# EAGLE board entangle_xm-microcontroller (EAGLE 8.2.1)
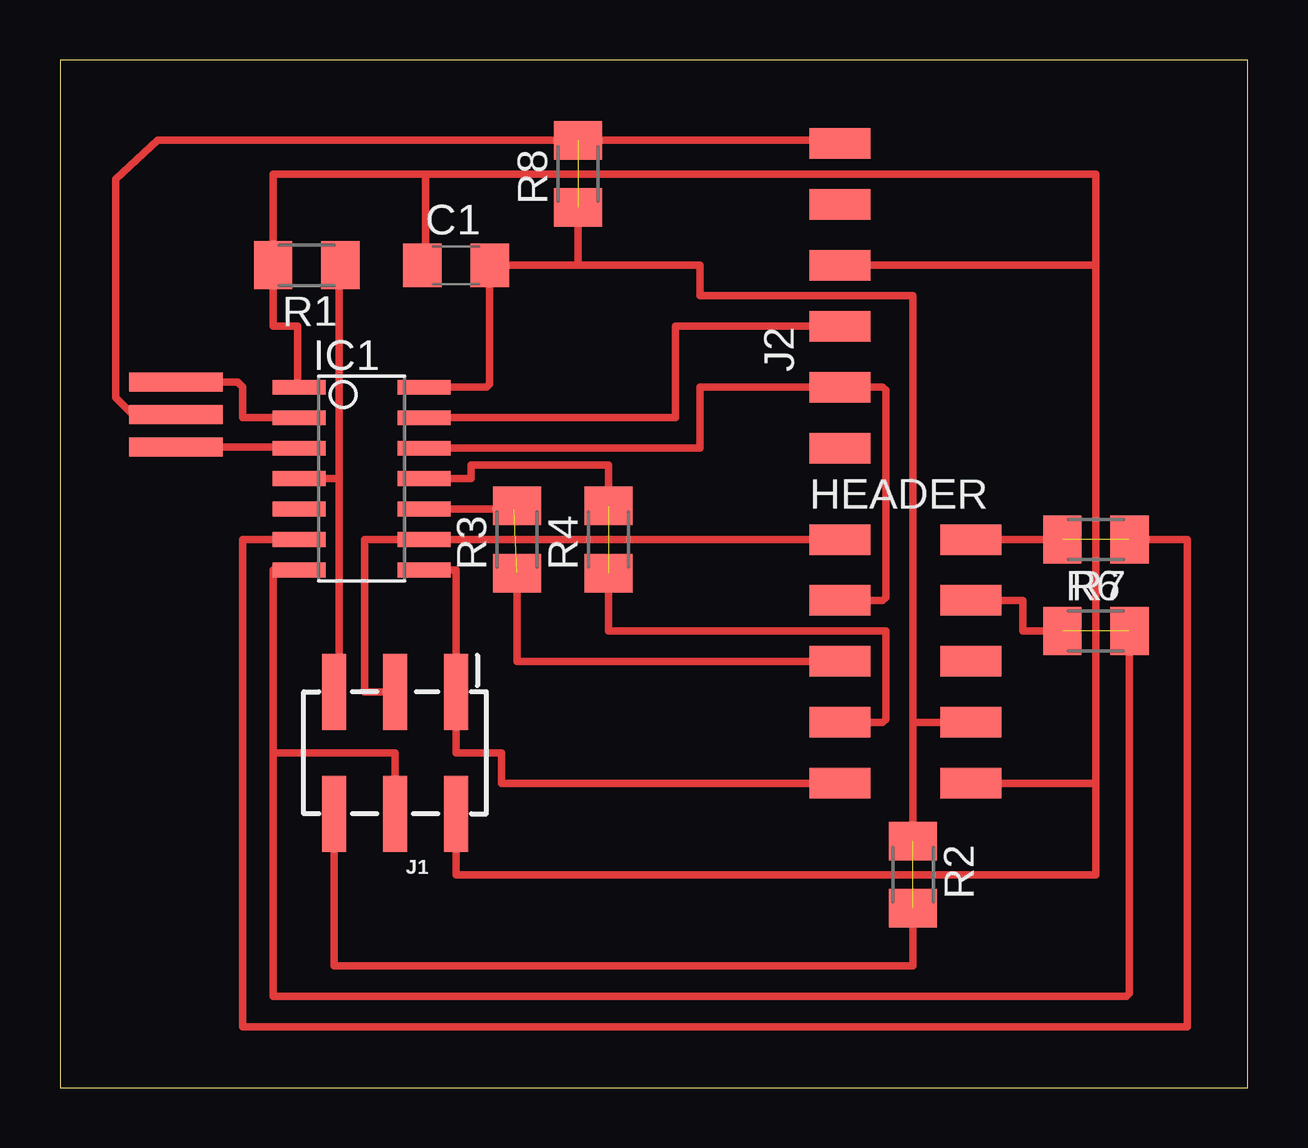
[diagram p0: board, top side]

Size 49.51 x 42.85 mm. Coordinates in mm from the lower left corner, seen from the top.
Outline: 0,0 49.51,0 49.51,42.85 0,42.85 0,0
Copper layers (1*16): Top 0.035mm / dielectric 1.5mm / Bottom 0.035mm
Design rules "default *": minimum track width 6mil, minimum drill 0.35mm, track to track 16mil, track to pad 16mil, pad to pad 16mil, via to via 16mil, smd to smd 16mil, copper to edge 40mil, drill to drill 6mil, minimum pad ring 10mil, minimum via ring 8mil, stop-mask expansion 4mil, vias tented up to drill 0mil, thermal gap 10mil

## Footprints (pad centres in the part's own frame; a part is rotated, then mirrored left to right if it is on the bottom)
C1206 = smd 1.6 x 1.8: 1 -1.4,0; 2 1.4,0
2X05SMD = smd 2.54 x 1.27: 1 -2.54,2.54; 2 2.92,2.54; 3 -2.54,0; 4 2.92,0; 5 -2.54,-2.54; 6 2.92,-2.54; 7 -2.54,-5.08; 8 2.92,-5.08; 9 -2.54,-7.62; 10 2.92,-7.62
SOIC14 = smd 0.61 x 2.21: 1 -3.81,-2.603; 2 -2.54,-2.603; 3 -1.27,-2.603; 4 0,-2.603; 5 1.27,-2.603; 6 2.54,-2.603; 7 3.81,-2.603; 8 3.81,2.603; 9 2.54,2.603; 10 1.27,2.603; 11 0,2.603; 12 -1.27,2.603; 13 -2.54,2.603; 14 -3.81,2.603
2X3_SMT_NO_POSTS = smd 1 x 3.17: 1 -2.54,-2.54; 2 -2.54,2.54; 3 0,-2.54; 4 0,2.54; 5 2.54,-2.54; 6 2.54,2.54
1X06SMD = smd 2.54 x 1.27: 1 0,6.35; 2 0,3.81; 3 0,1.27; 4 0,-1.27; 5 0,-3.81; 6 0,-6.35
M1206 = smd 1.6 x 2: 1 -1.4,0; 2 1.4,0
EFOBM = smd 0.8 x 3.9: 1 -1.35,0; 2 0,0; 3 1.35,0

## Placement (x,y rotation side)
C1  1uF  [C1206]  16.51,34.29 0 top
HEADER  PINHD-2X5-SMD  [2X05SMD]  35.05,20.32 0 top
IC1  ATTINY44-SSU  [SOIC14]  12.57,25.4 270 top
J1  [2X3_SMT_NO_POSTS]  13.97,13.97 180 top
J2  FTDI-SMD-HEADER  [1X06SMD]  32.51,33.02 0 top
R1  10k  [M1206]  10.29,34.29 180 top
R2  0  [M1206]  35.56,8.89 270 top
R3  0  [M1206]  19.05,22.86 90 top
R4  0  [M1206]  22.86,22.86 90 top
R6  0  [M1206]  43.18,19.05 0 top
R7  0  [M1206]  43.18,22.86 180 top
R8  0  [M1206]  21.59,38.1 90 top
XTAL1  20MHZ  [EFOBM]  4.83,28.07 270 top

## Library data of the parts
C1 R1-R4 R6-R8 = rcl
HEADER IC1 J2 XTAL1 = fab
J1 = SparkFun-Connectors

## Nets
CTS: J2.2
GND: C1.2 HEADER.8 IC1.14 J1.6 J2.1 R2.1 R2.2 R8.1 R8.2 XTAL1.2
MISO: HEADER.9 IC1.8 J1.1
MOSI: HEADER.4 IC1.7 J1.4 R6.1 R6.2
N/A: HEADER.6
PIN_A: HEADER.2 IC1.6 R7.1 R7.2
POT1: HEADER.5 IC1.10 R3.1 R3.2
POT3: HEADER.7 IC1.11 R4.1 R4.2
RST: IC1.4 J1.5 R1.1
RTS: J2.6
RXD: HEADER.3 IC1.12 J2.5
SCK: HEADER.1 IC1.9 J1.3
TXD: IC1.13 J2.4
VCC: C1.1 HEADER.10 IC1.1 J1.2 J2.3 R1.2
XTAL1: IC1.2 XTAL1.1
XTAL3: IC1.3 XTAL1.3

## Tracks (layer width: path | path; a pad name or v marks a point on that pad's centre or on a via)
GND  (2 unrouted)
  Top 0.305: 21.59,34.29 C1.2 17.91,29.34 17.78,29.21 IC1.14 | 21.59,34.29 R8.1 | 21.59,34.29 26.67,34.29 26.67,33.02 35.56,33.02 35.56,26.67 35.56,15.24 | HEADER.8 35.56,15.24 | 35.56,15.24 R2.1 | XTAL1.2 3.04,28.07 2.32,28.79 2.32,37.88 4.07,39.5 R8.2 32.64,39.5 32.76,39.63 33.02,39.37 J2.1 | R2.2 35.56,5.08 11.43,5.08 J1.6
MISO
  Top 0.305: IC1.8 16.51,21.59 J1.1 16.51,13.97 18.41,13.97 18.41,12.7 HEADER.9
MOSI  (1 unrouted)
  Top 0.305: 44.58,3.94 R6.2 | 44.58,3.94 44.45,3.81 | IC1.7 8.89,21.59 8.89,13.97 | 8.89,13.97 8.89,3.81 44.45,3.81 | 44.45,3.81 44.58,3.94 | 8.89,13.97 13.97,13.97 J1.4 | HEADER.4 40.13,20.32 40.13,19.05 R6.1
PIN_A  (1 unrouted)
  Top 0.305: HEADER.2 R7.2 | R7.1 46.99,22.86 46.99,2.54 7.62,2.54 7.62,22.86 IC1.6
POT1  (1 unrouted)
  Top 0.305: IC1.10 18.92,24.13 R3.2 | R3.1 19.05,17.78 HEADER.5
POT3  (1 unrouted)
  Top 0.305: IC1.11 17.14,25.4 17.14,25.96 22.86,25.96 R4.2 | R4.1 22.86,19.05 34.42,19.05 34.42,16.51 34.42,15.37 34.29,15.24 HEADER.7
RST
  Top 0.305: 11.63,25.6 11.63,25.4 | 11.63,25.4 11.63,16.71 J1.5 | IC1.4 11.63,25.4 | 11.63,25.4 11.63,34.24 R1.1
RXD
  Top 0.305: 28.57,29.21 29.21,29.21 | 29.21,29.21 J2.5 34.29,29.21 34.42,29.08 34.42,20.45 34.29,20.32 HEADER.3 | 29.21,29.21 26.67,29.21 26.67,26.67 IC1.12
SCK
  Top 0.305: HEADER.1 IC1.9 12.7,22.86 12.7,16.51 J1.3
TXD
  Top 0.305: IC1.13 25.65,27.94 25.65,31.75 J2.4
VCC
  Top 0.305: 15.24,38.1 15.24,34.42 C1.1 | 15.24,38.1 43.18,38.1 43.18,34.29 | 43.18,34.29 J2.3 | 43.18,12.7 43.18,34.29 | HEADER.10 43.18,12.7 | J1.2 16.51,8.89 43.18,8.89 43.18,12.7 | IC1.1 9.91,29.27 9.91,31.75 8.89,31.75 R1.2 8.89,38.1 15.24,38.1
XTAL1
  Top 0.305: XTAL1.1 7.41,29.42 7.62,29.21 7.62,27.94 IC1.2
XTAL3
  Top 0.305: XTAL1.3 9.92,26.72 IC1.3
